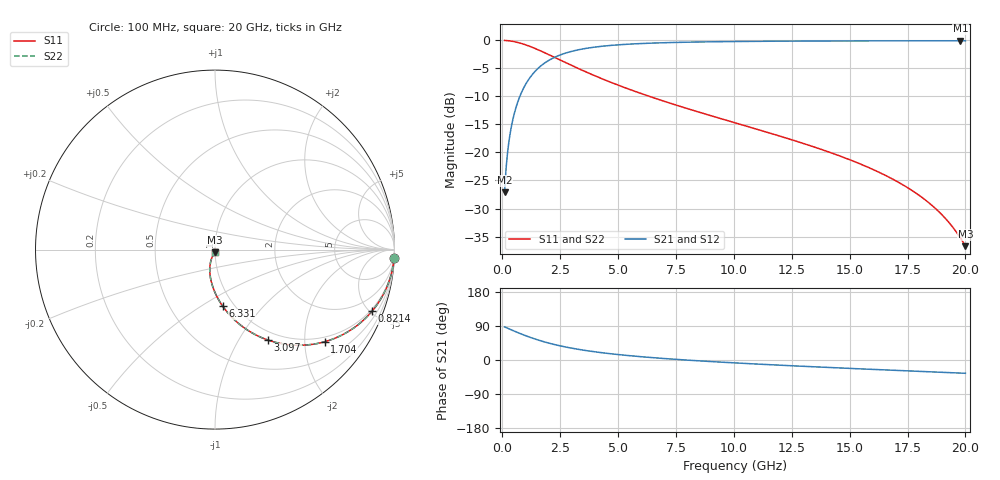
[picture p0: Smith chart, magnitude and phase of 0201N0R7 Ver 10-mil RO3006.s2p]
# GHz S MA R 50
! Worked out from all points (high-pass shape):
!   1601 points, 100 MHz to 20 GHz, reference 50 ohm
!   highest |S21| = -0.07 dB at 19.79 GHz (marker M1); lowest = -27.1 dB at 100 MHz (marker M2)
!   |S21| within 3 dB of the highest: 2.234 GHz to end of sweep
!   lowest |S11| = -36.7 dB at 20 GHz (marker M3), VSWR 1.03, Z = 49.8 - j1.44 ohm
!   |S11| at or under -10 dB: 6.361 GHz to end of sweep
!   |S22| runs from -36.7 to 0.0 dB; largest |S21 - S12| = 0
!   S11 on the Smith chart (normalised r, x): 100 MHz: 1, -42; 821.4 MHz: 0.87, -5.15; 1.704 GHz: 0.87, -2.47; 3.097 GHz: 0.88, -1.34; 6.331 GHz: 0.88, -0.62; 20 GHz: 1.00, -0.03
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0.1  0.999 -2.7  0.04397 87.3  0.04397 87.3  0.999 -2.7
0.2616875  0.9934 -7.1  0.1144 82.9  0.1144 82.9  0.9934 -7.1
0.3860625  0.9858 -10.4  0.1676 79.6  0.1676 79.6  0.9858 -10.4
0.572625  0.9695 -15.2  0.2445 74.8  0.2445 74.8  0.9695 -15.2
0.821375  0.94 -21.4  0.3402 68.6  0.3402 68.6  0.94 -21.4
1.206937  0.8821 -30.2  0.4696 59.7  0.4696 59.7  0.8821 -30.2
1.704438  0.7978 -40.1  0.6011 49.8  0.6011 49.8  0.7978 -40.1
2.400937  0.683 -51.1  0.728 38.7  0.728 38.7  0.683 -51.1
3.097437  0.5846 -59.6  0.8085 30.1  0.8085 30.1  0.5846 -59.6
3.420812  0.5451 -62.9  0.8353 26.8  0.8353 26.8  0.5451 -62.9
4.689438  0.4228 -73.1  0.9026 16.4  0.9026 16.4  0.4228 -73.1
6.331188  0.3178 -82.3  0.9439 7.0  0.9439 7.0  0.3178 -82.3
6.741625  0.2976 -84.2  0.9503 5.0  0.9503 5.0  0.2976 -84.2
10.05  0.184 -96.1  0.9777 -7.7  0.9777 -7.7  0.184 -96.1
13.37081  0.1137 -104.8  0.9875 -17.7  0.9875 -17.7  0.1137 -104.8
15.224  0.08268 -108.6  0.9902 -22.8  0.9902 -22.8  0.08268 -108.6
16.69162  0.06033 -110.6  0.9914 -26.6  0.9914 -26.6  0.06033 -110.6
17.68662  0.04592 -111.0  0.992 -29.2  0.992 -29.2  0.04592 -111.0
18.51994  0.03422 -110.0  0.9923 -31.3  0.9923 -31.3  0.03422 -110.0
19.21644  0.02471 -107.0  0.9924 -33.1  0.9924 -33.1  0.02471 -107.0
19.78856  0.01721 -100.7  0.9924 -34.5  0.9924 -34.5  0.01721 -100.7
20  0.01459 -96.4  0.9924 -35.0  0.9924 -35.0  0.01459 -96.4
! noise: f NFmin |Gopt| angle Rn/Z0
0.1  0.001071  0.9666  1.1  0.007268
2.301  0.005375  0.8277  5.233  0.00655
4.515  0.008293  0.7852  9.089  0.007886
6.729  0.01081  0.7584  12.99  0.008942
8.943  0.01311  0.7389  16.89  0.009841
11.14  0.01526  0.724  20.74  0.01063
13.36  0.01734  0.7122  24.58  0.01135
15.57  0.01935  0.7028  28.38  0.01202
17.79  0.02132  0.6953  32.13  0.01265
20  0.02326  0.6894  35.83  0.01324
